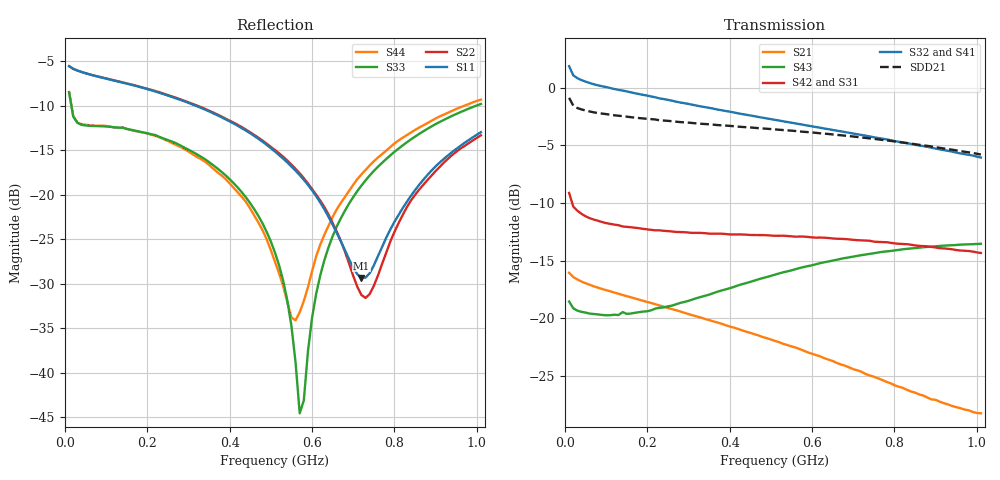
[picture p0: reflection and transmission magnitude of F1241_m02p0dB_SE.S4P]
! Integrated Device Technology
! Corporate Headquarters
! 6024 Silver Creek Valley Road
! San Jose, CA 95138  USA
! Phone:  1-408-284-8200
! Toll Free:  1-800-223-1366
! Webpage:  http://www.idt.com/
! Timing and RF Division
! 515 Groton Road, Suite 102
! Westford, MA 01886-6024
! Device:  F1241
! Description: Dual Intermediate Frequency Digital Variable Gain Amplifier
! Frequency:  10.0 -  500.00 MHz
! Package:  5x5 mm QFN Plastic Package: 32 pin
! Ports:  8 RF, 20 DC
!  Pin  1  = GA3  Pin 17  = RF OUT_B+
!  Pin  2  = GA4  Pin 18  = RF OUT_B-
!  Pin  3  = GA5  Pin 19  = STBY_B
!  Pin  4  = ISET_A  Pin 20  = Ground
!  Pin  5  = ISET_B  Pin 21  = Ground
!  Pin  6  = GB5  Pin 22  = STB_A
!  Pin  7  = GB4  Pin 23  = RF OUT_A-  = Port 4
!  Pin  8  = GB3  Pin 24  = RF OUT_A+  = Port 3
!  Pin  9  = GB2  Pin 25  = NO CONNECT
!  Pin 10  = GB1  Pin 26  = NO CONNECT
!  Pin 11  = RF IN_B+  Pin 27  = VCC
!  Pin 12  = RF IN_B-  Pin 28  = Ground
!  Pin 13  = Ground  Pin 29  = RF IN_A-  = Port 2
!  Pin 14  = VCC  Pin 30  = RF IN_A+  = Port 1
!  Pin 15  = NO CONNECT  Pin 31  = GA1
!  Pin 16  = NO CONNECT  Pin 32  = GA2
! State:  22
! Gain State:  -2.0 dB
! Voltages:  Vcc = +5.00 Volts  Icc approximately 160.0 mA or 80 mA per channel.
! Data:  The device was measured on a custom evaluation board which has
!  individual transmission lines to the RF pins.  Data was collected
!  using a calibrated network analyzer.  The evaluation board was
!  de-embedded using a port reference technique.
!  The reference plane is the edge of the package pin.
!  Only Channel A was measured.
!  This data is in single-ended operation.  If your needs are balanced
!  or differential S-parameters then this file needs to be used a
!  linear simulator.
! Misc:  Lot Code  160028MY
!  Action Tracker AT004
! Date Measured:  2014-08-14
! Date:  2014-08-28  MJV
! Note:
!  Integrated Device Technology supplies this data as a sample of measured
!  data at the package pin for this product.  Your particular data for this
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# Hz S dB R 50
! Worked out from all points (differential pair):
!   101 points, 10 MHz to 1.01 GHz, reference 50 ohm
!   strongest paths, dB at 10 MHz, 260 MHz, 510 MHz, 760 MHz, 1.01 GHz:
!     S32: 1.9, -1.1, -2.8, -4.3, -6.0
!     S41: 1.9, -1.1, -2.9, -4.5, -6.3
!     S42: -9.1, -12.5, -12.8, -13.4, -14.3
!     S31: -9.1, -12.5, -12.9, -13.5, -14.4
!     S43: -18.5, -18.9, -16.2, -14.3, -13.5
!     S21: -16.0, -19.2, -22.0, -25.2, -28.2
!   taken as a pair (ports 2,1 in; 3,4 out), SDD21 dB: -0.9, -2.9, -3.6, -4.5, -5.8
!   lowest |S11| = -29.3 dB at 720 MHz (marker M1), VSWR 1.07, Z = 47.9 - j2.58 ohm
!   |S11| at or under -10 dB: 317.4 MHz to end of sweep
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1e7  -5.57 -8.0  -16.04 -11.8  -35.00 -2.5  -22.98 8.7
     -16.05 -11.8  -5.56 -7.9  -23.01 8.4  -35.03 -2.0
     -9.12 157.2  1.88 169.0  -8.53 -39.3  -18.59 -179.1
     1.92 169.1  -9.12 157.3  -18.54 -179.1  -8.47 -39.1
4.5e8  -13.10 -39.2  -21.25 -38.8  -34.78 10.4  -23.99 -22.7
       -21.26 -39.2  -13.00 -35.7  -23.81 -22.4  -34.74 8.8
       -12.83 54.7  -2.40 115.4  -20.96 -24.7  -16.96 100.0
       -2.47 114.2  -12.77 54.0  -16.84 99.6  -21.56 -17.6
5.3e8  -15.95 -46.5  -22.14 -41.6  -34.02 9.8  -23.96 -26.9
       -22.22 -42.0  -15.74 -42.0  -23.68 -26.5  -34.01 7.8
       -12.94 40.0  -2.90 106.8  -29.68 -22.5  -16.16 88.5
       -3.00 105.5  -12.83 39.0  -16.00 88.3  -30.27 6.0
5.7e8  -17.80 -51.4  -22.62 -42.6  -33.65 9.1  -23.94 -28.9
       -22.67 -43.1  -17.59 -45.5  -23.64 -28.7  -33.59 7.1
       -13.01 33.2  -3.15 102.7  -44.53 28.2  -15.79 83.0
       -3.27 101.2  -12.91 32.2  -15.63 82.9  -33.19 74.7
6.3e8  -21.64 -62.6  -23.35 -43.8  -33.14 8.0  -23.96 -32.4
       -23.46 -44.3  -21.39 -55.0  -23.57 -32.1  -33.06 5.5
       -13.14 23.5  -3.53 96.5  -27.32 134.7  -15.31 75.0
       -3.67 95.0  -13.00 21.9  -15.13 74.8  -24.48 119.7
7.2e8  -29.33 -127.9  -24.52 -44.5  -32.32 5.2  -23.99 -37.4
       -24.64 -44.8  -31.26 -114.0  -23.54 -37.5  -32.29 2.6
       -13.36 10.1  -4.09 87.4  -18.96 135.0  -14.69 63.5
       -4.27 86.0  -13.23 8.2  -14.52 63.3  -17.71 126.8
1.01e9  -12.97 134.1  -28.08 -32.8  -30.38 -8.9  -24.60 -53.9
        -28.24 -31.6  -13.32 134.6  -23.81 -54.8  -30.26 -11.6
        -14.44 -24.4  -6.04 60.2  -9.81 124.3  -13.72 30.9
        -6.31 59.1  -14.33 -27.7  -13.53 30.8  -9.32 120.5
